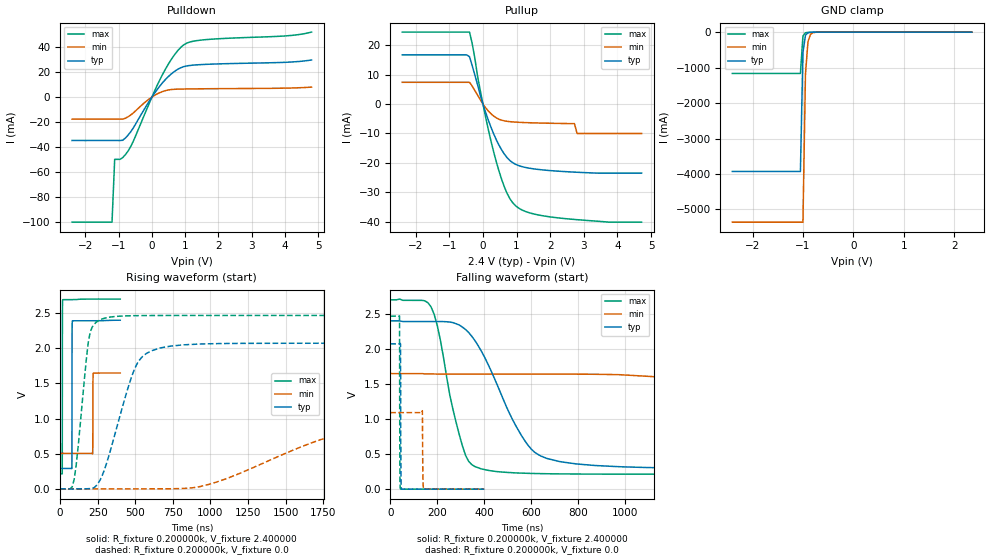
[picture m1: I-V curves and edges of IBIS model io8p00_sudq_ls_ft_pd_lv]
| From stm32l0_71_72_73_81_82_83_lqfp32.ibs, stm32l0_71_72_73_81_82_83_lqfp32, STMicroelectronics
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|   Model io8p00_sudq_ls_ft_pd_lv
[Model]  io8p00_sudq_ls_ft_pd_lv
Model_type I/O
Polarity   Non-Inverting
Enable   Active-Low
Vinl =   0.720000V
Vinh =   1.680000V
Vmeas =  1.200000V
Cref =   50.000000pF
Rref =   100.000000M
Vref =   0.0V
C_comp   2.317700pF   2.286600pF   2.332700pF
[Temperature Range]   25.000000   0.105000k   -40.000000
[Pullup Reference]   2.400000V   1.650000V   2.700000V
[Pulldown Reference]   0.0V   0.0V   0.0V
[POWER Clamp Reference]   2.400000V   1.650000V   2.700000V
[GND Clamp Reference]   0.0V   0.0V   0.0V
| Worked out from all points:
|   slope of the pulldown table from 0 to 0.36 V, typ, clamps not added: 28.4 ohm
|   slope of the pullup table from 0 to 0.36 V, typ, clamps not added: 32.2 ohm
|   GND clamp passes 1 mA (typ) near -0.64 V on its own axis
|   rising waveform, R_fixture 0.200000k, V_fixture 2.400000: 20-80 % time 640ps typ, 832ps min, 685ps max; typ from 0.29 V to 2.4 V
|   rising waveform, R_fixture 0.200000k, V_fixture 0.0: 20-80 % time 170ns typ, 823ns min, 66.7ns max; typ from 0 V to 2.07 V
|   falling waveform, R_fixture 0.200000k, V_fixture 2.400000: 20-80 % time 183ns typ, 736ns min, 91ns max; typ from 2.4 V to 0.29 V
|   falling waveform, R_fixture 0.200000k, V_fixture 0.0: 20-80 % time 1.11ns typ, 1.64ns min, 894ps max; typ from 2.07 V to 0 V
[Pulldown]
|Voltage   I(typ)   I(min)   I(max)
-2.4V     -34.71mA   -17.62mA   -100mA
-1.2V     -34.71mA   -17.62mA   -100mA
-1.12V    -34.71mA   -17.62mA   -49.77mA
-960mV    -34.71mA   -17.62mA   -49.77mA
-720mV    -30.52mA   -15.81mA   -43.23mA
-560mV    -24.66mA   -12.69mA   -35.3mA
-80mV     -3.3mA     -1.497mA   -4.982mA
320mV     11.47mA    4.39mA     18.08mA
640mV     19.72mA    6.139mA    32.34mA
960mV     24.33mA    6.432mA    41.77mA
1.52V     26.01mA    6.612mA    45.64mA
4.8V      29.64mA    7.944mA    51.92mA
[Pullup]
|Voltage   I(typ)   I(min)   I(max)
-2.4V     16.75mA    7.419mA    24.5mA
-400mV    16.1mA     7.419mA    24.5mA
-320mV    13.11mA    6.116mA    20.64mA
-160mV    6.589mA    3.049mA    9.467mA
80mV      -2.838mA   -1.261mA   -4.478mA
400mV     -12.2mA    -4.699mA   -19.76mA
720mV     -18.26mA   -5.869mA   -30.44mA
1.04V     -20.85mA   -6.184mA   -35.23mA
1.6V      -22.18mA   -6.425mA   -37.62mA
2.72V     -23.16mA   -6.64mA    -39.27mA
2.8V      -23.2mA    -10mA      -39.35mA
4.72V     -23.5mA    -10mA      -40.2mA
[GND_clamp]
|Voltage   I(typ)   I(min)   I(max)
-2.4V     -3.929A    -5.359A    -1.166A
-1.05V    -3.929A    -5.359A    -1.166A
-1V       -574.5mA   -5.359A    -109.1mA
-950mV    -90.03mA   -1.192A    -18.56mA
-900mV    -18.42mA   -269.7mA   -9.058mA
-850mV    -6.777mA   -63.61mA   -6.588mA
-800mV    -4.039mA   -16.67mA   -4.867mA
-650mV    -1.055mA   -1.235mA   -1.154mA
2.35V     52.69uA    50.02uA    36.84uA
[POWER_clamp]
|Voltage   I(typ)   I(min)   I(max)
-2.4V     0A         0A         0A
0V        0A         0A         0A
[Ramp]
| variable   typ   min   max
dV/dt_r  0.65004/0.30293u   0.18965/0.81904u   1.03746/0.14417u
dV/dt_f  0.75708/0.32433u   0.19722/0.85347u   1.13771/0.16150u
R_load = 50.000000
[Rising Waveform]
R_fixture= 0.200000k
V_fixture= 2.400000
V_fixture_min= 1.650000
V_fixture_max= 2.700000
|time   V(typ)   V(min)   V(max)
0s        290.5mV    505.1mV    212.9mV
14.01ns   290.5mV    505.1mV    219.9mV
15.22ns   290.5mV    505.1mV    2.491V
16.82ns   290.5mV    505.1mV    2.688V
77.68ns   288.7mV    505.1mV    2.691V
79.28ns   2.131V     505.1mV    2.691V
81.28ns   2.388V     505.1mV    2.691V
215.8ns   2.391V     497.2mV    2.699V
220.6ns   2.391V     1.644V     2.699V
400ns     2.399V     1.648V     2.699V
[Rising Waveform]
R_fixture= 0.200000k
V_fixture= 0.0
V_fixture_min= 0.0
V_fixture_max= 0.0
|time   V(typ)   V(min)   V(max)
0s        1.677nV    10.31nV    1.281nV
93.43ns   -107.7uV   10.31nV    137.3mV
200.2ns   3.627mV    10.31nV    2.232V
280.3ns   192.1mV    -22.87uV   2.417V
373.7ns   850mV      -23.01uV   2.453V
547.2ns   1.881V     273.3uV    2.464V
934.3ns   2.06V      34.38mV    2.466V
1.989us   2.071V     860.1mV    2.466V
2.789us   2.071V     1.055V     2.466V
13.33us   2.071V     1.091V     2.466V
[Falling Waveform]
R_fixture= 0.200000k
V_fixture= 2.400000
V_fixture_min= 1.650000
V_fixture_max= 2.700000
|time   V(typ)   V(min)   V(max)
0s        2.399V     1.648V     2.699V
173.5ns   2.389V     1.642V     2.599V
320.3ns   2.276V     1.64V      482.5mV
533.9ns   908mV      1.64V      231.8mV
640.6ns   473.2mV    1.64V      221.5mV
867.5ns   338.5mV    1.638V     214.8mV
1.361us   296.9mV    1.488V     213mV
2.229us   290.7mV    712.1mV    213mV
3.07us    290.5mV    543.2mV    213mV
13.33us   290.5mV    505.1mV    212.9mV
[Falling Waveform]
R_fixture= 0.200000k
V_fixture= 0.0
V_fixture_min= 0.0
V_fixture_max= 0.0
|time   V(typ)   V(min)   V(max)
0s        2.071V     1.091V     2.466V
39.24ns   2.071V     1.091V     2.47V
40.84ns   2.071V     1.091V     330.2mV
43.24ns   2.074V     1.091V     4.515mV
45.25ns   322.9mV    1.091V     262.9uV
48.05ns   2.769mV    1.091V     176.4uV
136.5ns   16.81uV    1.117V     133uV
138.9ns   16.9uV     193.5mV    132.6uV
142.5ns   17.03uV    3.471mV    131.9uV
400ns     1.677nV    10.31nV    1.281nV
